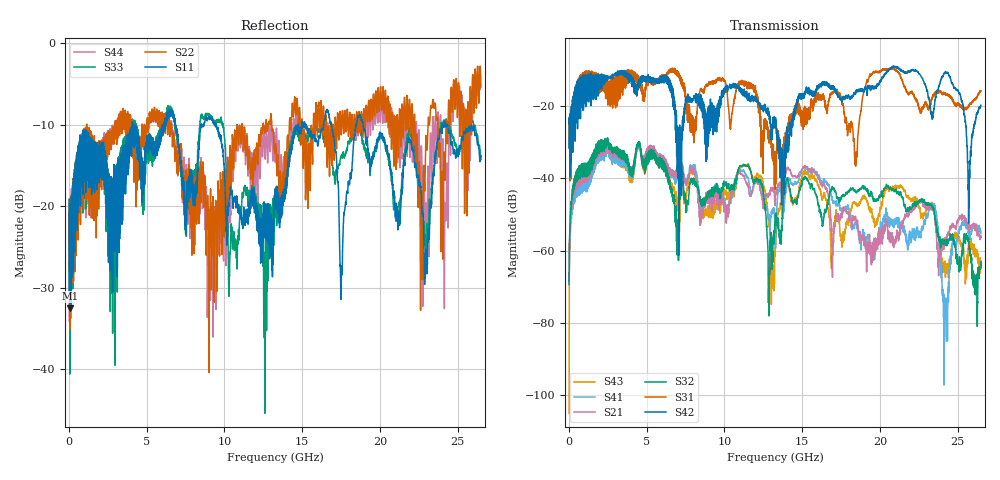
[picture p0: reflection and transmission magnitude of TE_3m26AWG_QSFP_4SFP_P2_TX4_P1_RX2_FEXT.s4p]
!Agilent Technologies,N5222A,MY51421691,A.10.00.00
!Agilent N5222A: A.10.00.00
!Date: Friday, January 30, 2015 12:36:48
!Correction: S11(Full 4 Port(1,2,3,4))
!S12(Full 4 Port(1,2,3,4))
!S13(Full 4 Port(1,2,3,4))
!S14(Full 4 Port(1,2,3,4))
!S21(Full 4 Port(1,2,3,4))
!S22(Full 4 Port(1,2,3,4))
!S23(Full 4 Port(1,2,3,4))
!S24(Full 4 Port(1,2,3,4))
!S31(Full 4 Port(1,2,3,4))
!S32(Full 4 Port(1,2,3,4))
!S33(Full 4 Port(1,2,3,4))
!S34(Full 4 Port(1,2,3,4))
!S41(Full 4 Port(1,2,3,4))
!S42(Full 4 Port(1,2,3,4))
!S43(Full 4 Port(1,2,3,4))
!S44(Full 4 Port(1,2,3,4))
!S4P File: Measurements: <S11,S12,S13,S14>,
!<S21,S22,S23,S24>,
!<S31,S32,S33,S34>,
!<S41,S42,S43,S44>:
# Hz S  dB  R 50.0
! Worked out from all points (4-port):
!   2650 points, 10 MHz to 26.5 GHz, reference 50 ohm
!   strongest paths, dB at 10 MHz, 6.63 GHz, 13.26 GHz, 19.88 GHz, 26.5 GHz:
!     S42: -24.8, -16.2, -25.3, -14.0, -19.8
!     S31: -24.9, -10.5, -43.1, -10.4, -15.7
!     S32: -69.3, -43.2, -53.1, -46.1, -63.0
!     S21: -69.3, -38.1, -47.6, -57.0, -56.0
!     S41: -69.5, -38.6, -54.9, -55.2, -55.3
!     S43: -104.9, -41.4, -60.3, -50.9, -64.6
!   lowest |S11| = -32.5 dB at 70 MHz (marker M1), VSWR 1.05, Z = 52.4 + j0.249 ohm
!   |S11| at or under -10 dB: start of sweep to 4.075 GHz; 9.454 GHz to 14.73 GHz (5.274 GHz wide, 43.6 % of centre); 18.91 GHz to 24.02 GHz (5.105 GHz wide, 23.8 % of centre)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
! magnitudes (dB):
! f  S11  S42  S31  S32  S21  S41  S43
! 10 MHz  -19.2  -24.8  -24.9  -69.3  -69.3  -69.5  -104.9
! 70 MHz  -32.5  -39.7  -40.8  -52.3  -54.9  -56.6  -54.8
! 4.47 GHz  -13.2  -15.1  -12.9  -30.1  -30.1  -31.1  -31.0
! 13.11 GHz  -22.7  -26.3  -30.5  -63.2  -43.3  -49.0  -64.1
! 23.44 GHz  -16.3  -21.7  -16.9  -48.0  -48.5  -47.0  -47.5
! 24.21 GHz  -9.7  -10.7  -16.6  -57.8  -56.3  -75.0  -65.9
! 26.5 GHz  -13.9  -19.8  -15.7  -63.0  -56.0  -55.3  -64.6
